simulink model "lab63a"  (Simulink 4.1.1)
settings: Solver=ode45  StartTime=0.0  StopTime=10.0  MaxStep=.01  RelTol=1e-6

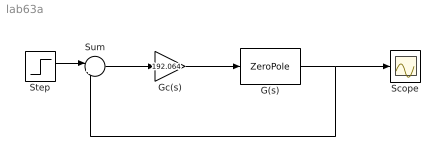
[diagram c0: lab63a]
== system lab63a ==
  G(s) : ZeroPole  Zeros=[]  Poles=[0 -6 -10]  Gain=[1]  AbsoluteTolerance=auto
  Gc(s) : Gain  Gain=192.064  Multiplication=Element-wise(K.*u)  SaturateOnIntegerOverflow=on
  Scope : Scope
  Step : Step  Time=1  Before=0  After=1  SampleTime=0
  Sum : Sum  Inputs=|+-  SaturateOnIntegerOverflow=on
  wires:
  Gc(s)/1 -> G(s)/1
  G(s)/1 -> Scope/1, Sum/2
  Sum/1 -> Gc(s)/1
  Step/1 -> Sum/1
